| IBIS file generated by GenIBIS323.exe Version 3.23
|   TDA2x
[IBIS ver]   5.0
[File name]   TDA2x.ibs
[File Rev]   1.3.3
[Date]   Fri Sep 20, 2013, 10:27:58
[Source]   Data created at Texas Instruments
[Notes]   TDA2x 17mm IBIS Model Revision History
   TDA2x Version 1.3.3, April 21, 2016
   - Created TDA2x version from parent device
   - Does not apply to TDA2Ex device
   Version 1.3.3, September 20, 2013
   - Updated the following models to more accurately
   represent the slew and delay characteristics.
   * Models include:
   > bc1833dv40dcpbfbhhvrxp1811_sscev
   > bc1833dv40dcpbfbp1811_ssceh
   > bc1833dv40dcpbfbp1811_sscev
   > bi2c1833dvfzp18_sscev
   > iq1833dvtckpbfbp18ll_sscev
   * Peripherals that use the corresponding IO buffers
   include:
   > GPMC
   > VIN/VOUT
   > MDIO
   > RGMII
   > UART
   > McASP
   > GPIO
   > MMC
   > SPI
   > DCAN
   > I2C
   > USB (AE6)
   > Debug
   > System and Misc Signals
   Version 1.3.2, August 14, 2013
   - Updated DDR models to address the minimum supply
   voltage and the discontinuities in the vertical
   single ended models.
   Version 1.3.1, August 5, 2013
   - Updated DDR2 (1.8V) models; regenerated at 400 MHz
   Version 1.3.0, June 14, 2013
   - Added I2C models
   - Added DDR Clock pins as differential
   Version 1.2.0, May 23, 2013
   - Added DDR2 (1.8V) models
   - Added DDR DQS pins as differential
   Version 1.1.1, April 8, 2013
   - Modifications, Additions, Deletions
   * Changed name of file to be package specific
   * Updated the following source IO models:
   > DDR_SEIOPB_V
   > DDR_SEIOPB_H
   > DDR_DIFFIOPB_H
   * Replaced the following source IO models:
   > GANGARX_HMAV10GS80 with GANGARX
   > SHANTANUTX_HMAV10GS80 with
   USB3_PCIEGEN1_PCIEGEN2_TX / SATATX
   * Added the following source IO models:
   > ACSPCIE_RX
   > IHHV1833DVHYP1811_SSCEV
   > BC1833DV40DCPBFBHHVRXP1811_SSCEV
   > IQ1833DVTCKPBFBP18LL_SSCEV
   * Updated the RLC data for all pins
   * Changed the supported DDR voltage from 1.2V/1.5V
   to 1.35/1.5V for DDR3 usage
   * Updated the ball number for some signals
   Version 1.0, December 4, 2012
   - Initial Release
   Note 1) Checked by IBISCHK5.
   Note 2) Interfaces Included in this IBIS Model
   - DDR1
   - GPMC
   - VIP1
   - VIP2
   - DSS
   - HDMI1
   - RGMII
   - UART3
   - USB1
   - PCIE
   - XREFCLK
   - McASP1,2,3,4,5
   - MMC3
   - SPI1,2
   - DCAN
   - UART1,2
   - SATA1
   - I2C1
   - I2C2
[Disclaimer] Please be aware that in the absence of a written agreement,
   Texas Instruments (TI) assumes no liability for: 1) the
   accuracy of the IBIS models provided to your company, 2) the
   proper functioning of these IBIS models in your design or for
   any resulting applications, or, 3) infringement of patents,
   copyrights, or intellectual property rights resulting from
   your use of these IBIS models. TI provides IBIS models as a
   service to our customers and therefore reserves the right to
   limit distribution of the IBIS models.
[Copyright]   Property of Texas Instruments Incorporated. Unauthorised
   reproduction and/or distribution is strictly prohibited. This
   product is protected under copyright law and trade secret law
   as an unpublished work. Created 2013,(C) Copyright 2013,
   Texas Instruments Incorporated., All Rights Reserved. These
   commodities are under the U.S. Government distribution license
   control.As such,they are not to be re-exported without the
   prior approval of the U.S. Department of Commerce.
|   Component TDA2x
[Component]   TDA2x
[Manufacturer]   Texas Instruments.
| Source IO level model revisions
|Model   Revision   Date
|DDR_SEIOPB_V   2.4   14 Aug 2013
|BC1833DV40DCPBFBP1811_SSCEH   2.0   Sep 11, 2013
|DDR_SEIOPB_H   2.4   14 Aug 2013
|GANGARX   1   Sep 04, 2012
|DDR_DIFFIOPB_H   2.4   14 Aug 2013
|IQ1833DVTCKPBFBP18LL_SSCEV   2.0   Sep 11, 2013
|HDMITXPHY   0.8   Jul 12, 2011
|USB3_PCIEGEN1_PCIEGEN2_TX   1.0   Nov 07, 2012
|ACSPCIE_RX   0.5   May 16, 2012
|DDR_DIFFIOPB_V   2.4   14 Aug 2013
|BI2C1833DVFZP18_SSCEV   2.0   Sep 11, 2013
|USB2PHYCORE_HMAV10GS80   0.8   July 13, 2011
|BC1833DV40DCPBFBP1811_SSCEV   2.0   Sep 11, 2013
|BC1833DV40DCPBFBHHVRXP1811_SSCEV   2.0   Sep 11, 2013
|IHHV1833DVHYP1811_SSCEV   1.0   Dec 24, 2012
[Package]
|   typ   min   max
R_pkg   0.451804411428571   26.877E-3   1221.700E-3
L_pkg   2.34772857142857E-009 0.659E-9   5.652E-9
C_pkg   1.16282285714286E-012 0.592E-12   2.087E-12
[Pin]   signal_name   model_name   R_pin   L_pin   C_pin
Y7   ATESTV   NC
E21   DCAN1_RX   Selector_16  463.710E-3 2.345E-9   1.144E-12
E19   DCAN1_TX   Selector_16  130.950E-3 0.880E-9   0.804E-12
AC20   DDR1_A5   Selector_2   601.780E-3 2.409E-9   1.006E-12
M21   DDR1_D30   Selector_15  445.880E-3 2.447E-9   1.330E-12
P24   DDR1_DQSN3   Selector_13  461.360E-3 2.464E-9   1.164E-12
P22   DDR1_D29   Selector_15  493.080E-3 2.118E-9   1.140E-12
T24   DDR1_DQM2   Selector_17  425.130E-3 2.082E-9   1.136E-12
P21   DDR1_DQM3   Selector_17  341.520E-3 1.786E-9   1.246E-12
T25   DDR1_D23   Selector_15  416.820E-3 2.054E-9   1.079E-12
Y21   DDR1_D0   Selector_15  391.590E-3 1.635E-9   0.982E-12
U25   DDR1_DQS2   Selector_5   365.560E-3 2.080E-9   1.161E-12
R22   DDR1_D16   Selector_15  408.140E-3 2.006E-9   1.164E-12
V24   DDR1_DQSN1   Selector_13  332.830E-3 1.926E-9   1.098E-12
M25   DDR1_ECC_D0   Selector_15  615.370E-3 2.868E-9   1.361E-12
P23   DDR1_D17   Selector_15  376.150E-3 1.866E-9   1.181E-12
N24   DDR1_D26   Selector_15  465.800E-3 2.306E-9   1.305E-12
AE23   DDR1_BA2   Selector_2   668.110E-3 3.078E-9   1.348E-12
AD18   DDR1_A15   Selector_2   645.490E-3 2.726E-9   1.063E-12
AA25   DDR1_DQS0   Selector_5   355.560E-3 2.004E-9   1.041E-12
V23   DDR1_D11   Selector_15  378.670E-3 1.867E-9   1.016E-12
AD21   DDR1_WEN   Selector_2   660.220E-3 2.763E-9   1.137E-12
AC18   DDR1_CASN   Selector_2   579.300E-3 2.239E-9   1.179E-12
K23   DDR1_ECC_D4   Selector_15  623.560E-3 2.738E-9   1.233E-12
AA22   DDR1_D6   Selector_15  394.470E-3 1.827E-9   1.021E-12
AE20   DDR1_A1   Selector_2   532.570E-3 2.267E-9   1.397E-12
Y25   DDR1_D5   Selector_15  383.930E-3 2.024E-9   1.076E-12
AC21   DDR1_A4   Selector_2   645.850E-3 2.449E-9   1.255E-12
AA19   DDR1_A7   Selector_2   497.700E-3 2.270E-9   1.061E-12
R24   DDR1_D20   Selector_15  418.610E-3 2.097E-9   1.085E-12
M22   DDR1_D27   Selector_15  447.080E-3 2.390E-9   1.268E-12
K24   DDR1_DQSN_ECC   Selector_13  564.990E-3 2.914E-9   1.394E-12
AC22   DDR1_CSN0   Selector_2   637.030E-3 2.509E-9   1.304E-12
L25   DDR1_ECC_D6   Selector_15  641.400E-3 3.008E-9   1.214E-12
V22   DDR1_D12   Selector_15  385.360E-3 1.662E-9   1.016E-12
J23   DDR1_ECC_D2   Selector_15  644.370E-3 3.012E-9   1.390E-12
W22   DDR1_D9   Selector_15  388.130E-3 1.861E-9   0.929E-12
L24   DDR1_ECC_D5   Selector_15  616.230E-3 2.846E-9   1.348E-12
AA20   DDR1_DQM0   Selector_17  308.850E-3 1.445E-9   1.026E-12
AB24   DDR1_A12   Selector_2   640.730E-3 2.440E-9   1.311E-12
AB21   DDR1_VREF0   NC
AB20   DDR1_A8   Selector_2   621.390E-3 2.157E-9   1.190E-12
M24   DDR1_ECC_D1   Selector_15  635.500E-3 2.924E-9   1.360E-12
P25   DDR1_DQS3   Selector_5   465.950E-3 2.482E-9   1.310E-12
AE19   DDR1_RASN   Selector_2   604.870E-3 2.186E-9   1.440E-12
AC25   DDR1_CK   Selector_14  654.810E-3 2.979E-9   1.334E-12
U24   DDR1_DQSN2   Selector_13  347.950E-3 1.962E-9   1.148E-12
V21   DDR1_D13   Selector_15  172.230E-3 1.807E-9   1.120E-12
Y22   DDR1_D3   Selector_15  389.570E-3 1.662E-9   0.972E-12
AC23   DDR1_A6   Selector_2   646.310E-3 2.733E-9   1.343E-12
W25   DDR1_D4   Selector_15  390.500E-3 2.069E-9   1.038E-12
N22   DDR1_D31   Selector_15  439.830E-3 2.016E-9   1.110E-12
AA18   DDR1_A3   Selector_2   488.480E-3 2.281E-9   1.285E-12
N23   DDR1_D28   Selector_15  483.920E-3 2.290E-9   1.115E-12
K25   DDR1_DQS_ECC   Selector_5   573.180E-3 2.913E-9   1.379E-12
N21   DDR1_D24   Selector_15  459.010E-3 2.201E-9   1.173E-12
R25   DDR1_D19   Selector_15  417.700E-3 2.100E-9   1.051E-12
AA21   DDR1_D7   Selector_15  371.740E-3 1.559E-9   1.031E-12
AD17   DDR1_A13   Selector_2   609.270E-3 2.349E-9   1.196E-12
W21   DDR1_D8   Selector_15  394.160E-3 1.752E-9   1.125E-12
AE21   DDR1_BA1   Selector_2   642.880E-3 2.917E-9   1.281E-12
U21   DDR1_DQM1   Selector_17  274.990E-3 1.700E-9   1.008E-12
R21   DDR1_D21   Selector_15  361.860E-3 2.148E-9   1.166E-12
W24   DDR1_D2   Selector_15  385.490E-3 2.016E-9   1.030E-12
AC24   DDR1_NCK   Selector_9   652.970E-3 3.000E-9   1.347E-12
AB18   DDR1_A0   Selector_2   507.480E-3 2.394E-9   1.329E-12
AB25   DDR1_A11   Selector_2   632.080E-3 2.629E-9   1.369E-12
K22   DDR1_DQM_ECC   Selector_17  636.180E-3 2.670E-9   1.250E-12
AE17   DDR1_A14   Selector_2   619.970E-3 2.435E-9   1.045E-12
AA24   DDR1_DQSN0   Selector_13  350.870E-3 2.011E-9   0.956E-12
AD23   DDR1_ODT0   Selector_2   709.530E-3 3.055E-9   1.355E-12
N25   DDR1_D25   Selector_15  493.150E-3 2.453E-9   1.182E-12
U23   DDR1_D14   Selector_15  332.810E-3 1.858E-9   1.148E-12
AD24   DDR1_A2   Selector_2   664.380E-3 3.045E-9   1.281E-12
AB23   DDR1_A9   Selector_2   638.160E-3 2.413E-9   1.190E-12
U22   DDR1_D15   Selector_15  331.540E-3 1.705E-9   1.154E-12
T22   DDR1_D22   Selector_15  387.150E-3 1.754E-9   1.063E-12
AE18   DDR1_BA0   Selector_2   627.580E-3 2.515E-9   1.321E-12
L22   DDR1_ECC_D3   Selector_15  622.650E-3 2.631E-9   1.356E-12
T21   DDR1_D18   Selector_15  310.240E-3 1.491E-9   0.938E-12
Y24   DDR1_D1   Selector_15  379.970E-3 1.917E-9   0.986E-12
L21   DDR1_ECC_D7   Selector_15  683.310E-3 2.897E-9   1.313E-12
AB19   DDR1_CKE   Selector_2   540.190E-3 2.206E-9   0.997E-12
V25   DDR1_DQS1   Selector_5   331.770E-3 1.853E-9   1.187E-12
AB22   DDR1_A10   Selector_2   630.700E-3 2.135E-9   1.277E-12
AD20   DDR1_RST   Selector_2   668.060E-3 2.685E-9   1.312E-12
W23   DDR1_D10   Selector_15  362.420E-3 1.740E-9   0.960E-12
E20   EMU0   Selector_16  277.650E-3 1.610E-9   1.063E-12
D21   EMU1   Selector_16  479.230E-3 2.366E-9   1.180E-12
Y1   GPIO6_10   Selector_10  521.740E-3 3.084E-9   1.420E-12
W1   GPIO6_11   Selector_10  433.870E-3 2.183E-9   1.101E-12
E2   GPMC_A24   Selector_10  359.070E-3 1.975E-9   1.131E-12
D1   GPMC_A22   Selector_10  421.510E-3 2.285E-9   1.160E-12
G3   GPMC_AD9   Selector_10  421.090E-3 2.287E-9   1.339E-12
G2   GPMC_AD8   Selector_10  267.490E-3 1.834E-9   1.032E-12
N2   GPMC_A4   Selector_10  371.530E-3 2.027E-9   1.129E-12
G1   GPMC_AD2   Selector_10  320.320E-3 2.077E-9   1.172E-12
F5   GPMC_AD13   Selector_10  123.700E-3 0.854E-9   0.834E-12
K6   GPMC_A17   Selector_10  215.800E-3 1.496E-9   1.086E-12
N3   GPMC_A0   Selector_10  245.300E-3 1.481E-9   1.066E-12
L4   GPMC_A13   Selector_10  257.060E-3 1.520E-9   0.935E-12
D3   GPMC_A20   Selector_10  266.870E-3 1.817E-9   1.157E-12
M4   GPMC_A7   Selector_10  227.660E-3 1.435E-9   0.941E-12
K2   GPMC_CS3   Selector_10  402.200E-3 2.063E-9   1.291E-12
F3   GPMC_A27   Selector_10  577.110E-3 3.342E-9   1.515E-12
H4   GPMC_AD5   Selector_10  387.900E-3 2.353E-9   1.054E-12
P3   GPMC_A1   Selector_10  400.770E-3 2.018E-9   1.094E-12
L5   GPMC_A12   Selector_10  197.850E-3 1.267E-9   0.949E-12
H2   GPMC_AD3   Selector_10  184.450E-3 1.453E-9   0.953E-12
G4   GPMC_AD10   Selector_10  472.420E-3 2.631E-9   1.296E-12
H3   GPMC_AD4   Selector_10  481.420E-3 2.604E-9   1.345E-12
J3   GPMC_BEN1   Selector_10  422.980E-3 2.428E-9   1.285E-12
M5   GPMC_A6   Selector_10  230.850E-3 1.431E-9   0.974E-12
M3   GPMC_A9   Selector_10  349.820E-3 1.861E-9   0.942E-12
M6   GPMC_A10   Selector_10  290.780E-3 2.115E-9   1.176E-12
E3   GPMC_A25   Selector_10  523.900E-3 2.967E-9   1.440E-12
H6   GPMC_AD1   Selector_10  70.140E-3  0.745E-9   0.738E-12
K5   GPMC_A18   Selector_10  147.480E-3 0.958E-9   0.983E-12
M2   GPMC_BEN0   Selector_10  384.550E-3 1.923E-9   0.985E-12
J4   GPMC_AD0   Selector_10  445.610E-3 2.363E-9   1.292E-12
E5   GPMC_AD14   Selector_10  198.000E-3 1.413E-9   0.933E-12
K4   GPMC_CS0   Selector_10  246.530E-3 1.417E-9   0.920E-12
G5   GPMC_AD11   Selector_10  110.560E-3 0.844E-9   0.779E-12
G6   GPMC_AD12   Selector_10  126.070E-3 1.000E-9   0.784E-12
P1   GPMC_A2   Selector_10  533.070E-3 2.610E-9   1.250E-12
F4   GPMC_AD15   Selector_10  279.360E-3 1.630E-9   1.008E-12
L3   GPMC_A14   Selector_10  286.770E-3 1.587E-9   1.026E-12
C1   GPMC_CS1   Selector_10  425.990E-3 2.291E-9   1.117E-12
L2   GPMC_A15   Selector_10  427.460E-3 2.176E-9   1.188E-12
J5   GPMC_ADVN_ALE   Selector_10  126.710E-3 0.981E-9   0.885E-12
K1   GPMC_WAIT0   Selector_10  400.740E-3 2.102E-9   1.063E-12
D2   GPMC_A21   Selector_10  328.920E-3 1.891E-9   1.266E-12
P2   GPMC_A3   Selector_10  430.140E-3 2.168E-9   1.183E-12
E1   GPMC_A23   Selector_10  416.150E-3 2.285E-9   1.208E-12
L1   GPMC_A16   Selector_10  402.630E-3 2.104E-9   1.132E-12
M1   GPMC_A8   Selector_10  488.790E-3 2.415E-9   1.239E-12
C2   GPMC_A19   Selector_10  444.750E-3 2.652E-9   1.312E-12
F2   GPMC_WEN   Selector_10  424.150E-3 3.038E-9   1.497E-12
N6   GPMC_CLK   Selector_10  302.950E-3 1.983E-9   1.157E-12
N1   GPMC_A5   Selector_10  468.120E-3 2.440E-9   1.222E-12
E4   GPMC_A26   Selector_10  191.540E-3 1.238E-9   0.848E-12
N5   GPMC_A11   Selector_10  295.970E-3 1.733E-9   1.034E-12
H5   GPMC_AD6   Selector_10  131.890E-3 0.963E-9   0.816E-12
F1   GPMC_AD7   Selector_10  297.000E-3 1.814E-9   1.142E-12
H1   GPMC_OEN_REN   Selector_10  233.470E-3 1.955E-9   1.147E-12
K3   GPMC_CS2   Selector_10  263.620E-3 1.512E-9   0.947E-12
AE13   HDMI1_CLOCKY   Model_499   511.060E-3 3.576E-9   0.726E-12
AE14   HDMI1_DATA0Y   Model_499   449.700E-3 3.320E-9   0.646E-12
AE16   HDMI1_DATA2Y   Model_499   470.780E-3 3.387E-9   0.653E-12
AD14   HDMI1_DATA0X   Model_498   449.260E-3 3.078E-9   0.741E-12
AD16   HDMI1_DATA2X   Model_498   450.890E-3 2.959E-9   0.592E-12
AD15   HDMI1_DATA1X   Model_498   425.260E-3 2.890E-9   0.667E-12
AE15   HDMI1_DATA1Y   Model_499   463.320E-3 3.318E-9   0.738E-12
AD13   HDMI1_CLOCKX   Model_498   503.180E-3 3.217E-9   0.705E-12
G25   I2C1_SDA   Selector_7   984.150E-3 4.471E-9   1.624E-12
F23   I2C2_SCL   Selector_7   892.510E-3 3.917E-9   1.539E-12
G24   I2C1_SCL   Selector_7   1020.300E-3 4.477E-9   1.684E-12
F22   I2C2_SDA   Selector_7   802.230E-3 3.606E-9   1.632E-12
AE12   LJCB_CLKP   Model_699   427.270E-3 2.549E-9   0.759E-12
AD12   LJCB_CLKN   Model_699   399.560E-3 2.285E-9   0.821E-12
A17   MCASP1_AXR9   Selector_16  639.010E-3 3.067E-9   1.257E-12
B24   MCASP1_FSX   Selector_16  1110.900E-3 4.998E-9   1.700E-12
B15   MCASP1_AXR0   Selector_16  422.670E-3 2.198E-9   1.107E-12
C15   MCASP1_AXR14   Selector_16  253.340E-3 1.565E-9   0.933E-12
A23   MCASP1_AXR13   Selector_16  1092.300E-3 4.982E-9   1.540E-12
A15   MCASP1_AXR1   Selector_16  523.880E-3 2.560E-9   1.051E-12
A19   MCASP1_AXR10   Selector_16  779.980E-3 3.618E-9   1.389E-12
A21   MCASP1_AXR12   Selector_16  895.110E-3 4.149E-9   1.564E-12
B16   MCASP1_AXR15   Selector_16  466.140E-3 2.322E-9   1.195E-12
A16   MCASP1_AXR8   Selector_16  466.300E-3 2.392E-9   1.090E-12
A20   MCASP1_AXR11   Selector_16  890.820E-3 4.087E-9   1.607E-12
C25   MCASP1_ACLKX   Selector_16  1221.700E-3 5.206E-9   1.867E-12
B17   MCASP2_AXR3   Selector_16  518.380E-3 2.575E-9   1.145E-12
B21   MCASP2_ACLKX   Selector_16  767.630E-3 3.690E-9   1.542E-12
B20   MCASP2_FSX   Selector_16  704.240E-3 3.331E-9   1.350E-12
B23   MCASP2_AXR2   Selector_16  986.210E-3 4.307E-9   1.727E-12
C16   MCASP3_FSX   Selector_16  342.390E-3 1.864E-9   1.011E-12
C20   MCASP3_AXR1   Selector_16  742.080E-3 3.602E-9   1.505E-12
C17   MCASP3_AXR0   Selector_16  324.500E-3 1.806E-9   1.002E-12
B19   MCASP3_ACLKX   Selector_16  543.620E-3 2.687E-9   1.100E-12
D23   MCASP4_FSX   Selector_16  953.700E-3 4.218E-9   1.664E-12
E23   MCASP4_AXR1   Selector_16  1178.700E-3 5.214E-9   2.087E-12
E24   MCASP4_ACLKX   Selector_16  1218.800E-3 5.203E-9   2.019E-12
E25   MCASP4_AXR0   Selector_16  1064.300E-3 4.828E-9   1.872E-12
V2   MCASP5_AXR0   Selector_10  501.640E-3 2.583E-9   1.207E-12
W2   MCASP5_FSX   Selector_10  394.660E-3 2.073E-9   1.152E-12
V1   MCASP5_ACLKX   Selector_10  499.360E-3 2.696E-9   1.265E-12
U1   MCASP5_AXR1   Selector_10  329.480E-3 1.886E-9   1.111E-12
T1   MDIO_D   Selector_10  487.610E-3 2.629E-9   1.329E-12
R3   MDIO_MCLK   Selector_10  634.770E-3 3.175E-9   1.417E-12
W4   MMC3_CMD   Selector_10  380.060E-3 2.037E-9   1.208E-12
U5   MMC3_DAT2   Selector_10  174.080E-3 1.188E-9   1.065E-12
U6   MMC3_DAT0   Selector_10  45.368E-3  0.707E-9   0.758E-12
W3   MMC3_DAT6   Selector_10  534.640E-3 3.025E-9   1.596E-12
V3   MMC3_DAT3   Selector_10  556.770E-3 3.106E-9   1.485E-12
V4   MMC3_DAT7   Selector_10  212.570E-3 1.339E-9   0.912E-12
V6   MMC3_DAT1   Selector_10  176.740E-3 1.110E-9   1.078E-12
W5   MMC3_CLK   Selector_10  330.100E-3 2.088E-9   1.282E-12
W6   MMC3_DAT5   Selector_10  334.710E-3 2.207E-9   1.268E-12
V5   MMC3_DAT4   Selector_10  246.460E-3 1.514E-9   0.871E-12
G22   NMIN   Selector_6   798.970E-3 3.586E-9   1.571E-12
AA11   ON_OFF   Selector_18  111.570E-3 1.030E-9   0.880E-12
AE11   PCIE_TXP0   Selector_12  465.680E-3 2.523E-9   0.681E-12
AD10   PCIE_RXN0   Model_332   460.180E-3 2.608E-9   0.752E-12
AE10   PCIE_RXP0   Model_332   452.350E-3 2.692E-9   0.773E-12
AD11   PCIE_TXN0   Selector_8   456.230E-3 2.425E-9   0.719E-12
F17   PORZ   Selector_19  38.459E-3  0.727E-9   0.775E-12
H21   RESETN   Selector_6   766.440E-3 3.519E-9   1.404E-12
U3   RGMII0_RXCTL   Selector_10  399.210E-3 2.120E-9   1.010E-12
P5   RGMII0_RXD3   Selector_10  207.740E-3 1.332E-9   0.983E-12
U2   RGMII0_RXC   Selector_10  486.610E-3 2.421E-9   1.222E-12
T4   RGMII0_TXD1   Selector_10  305.720E-3 1.692E-9   1.003E-12
R6   RGMII0_TXC   Selector_10  145.130E-3 1.121E-9   0.891E-12
U4   RGMII0_RXD2   Selector_10  554.050E-3 2.804E-9   1.434E-12
T3   RGMII0_RXD1   Selector_10  465.860E-3 2.261E-9   1.169E-12
R5   RGMII0_TXD0   Selector_10  208.370E-3 1.336E-9   0.932E-12
T6   RGMII0_TXD2   Selector_10  267.640E-3 1.638E-9   1.041E-12
P6   RGMII0_TXCTL   Selector_10  33.356E-3  0.703E-9   0.782E-12
R4   RGMII0_RXD0   Selector_10  355.120E-3 1.850E-9   0.933E-12
T5   RGMII0_TXD3   Selector_10  276.180E-3 1.590E-9   1.014E-12
R2   RMII_MHZ_50_CLK   Selector_10  556.030E-3 2.883E-9   1.357E-12
G21   RSTOUTN   Selector_1   554.330E-3 2.837E-9   1.368E-12
AA13   RTC_OSC_XI_CLKIN32   NC
AA10   RTC_PORZ   Selector_19  154.820E-3 1.596E-9   1.057E-12
AA12   RTC_OSC_XO   NC
AA9   RTC_ISO   Selector_19  204.150E-3 1.944E-9   1.014E-12
D19   RTCK   Selector_1   335.270E-3 1.806E-9   1.055E-12
D22   SPI1_CS0   Selector_16  760.230E-3 3.397E-9   1.508E-12
E22   SPI1_D0   Selector_16  841.460E-3 3.816E-9   1.670E-12
C18   SPI1_SCLK   Selector_16  306.460E-3 1.707E-9   1.003E-12
C21   SPI1_D1   Selector_16  643.920E-3 2.923E-9   1.380E-12
D16   SPI1_CS1   Selector_16  220.460E-3 1.333E-9   0.935E-12
C24   SPI1_CS3   Selector_16  870.640E-3 4.054E-9   1.515E-12
C19   SPI1_CS2   Selector_16  373.120E-3 1.985E-9   1.089E-12
F25   SPI2_D1   Selector_16  1044.700E-3 4.580E-9   1.674E-12
E16   SPI2_D0   Selector_16  27.015E-3  0.667E-9   0.744E-12
D17   SPI2_CS0   Selector_16  138.970E-3 1.020E-9   0.852E-12
F24   SPI2_SCLK   Selector_16  1000.600E-3 4.289E-9   1.702E-12
E18   TCLK   Selector_3   153.370E-3 1.082E-9   0.951E-12
D20   TDI   Selector_6   384.220E-3 1.963E-9   1.093E-12
F21   TDO   Selector_1   634.310E-3 3.028E-9   1.308E-12
D18   TMS   Selector_6   152.740E-3 1.022E-9   0.961E-12
E17   TRSTN   Selector_6   26.877E-3  0.659E-9   0.750E-12
H24   UART1_RTSN   Selector_16  849.610E-3 3.946E-9   1.646E-12
H22   UART1_TXD   Selector_16  758.590E-3 3.574E-9   1.466E-12
G23   UART1_RXD   Selector_16  780.640E-3 3.621E-9   1.564E-12
H25   UART1_CTSN   Selector_16  914.490E-3 4.170E-9   1.617E-12
J24   UART2_RTSN   Selector_16  830.410E-3 3.662E-9   1.506E-12
J22   UART2_CTSN   Selector_16  648.420E-3 2.921E-9   1.361E-12
H23   UART2_RXD   Selector_16  725.070E-3 3.286E-9   1.376E-12
J25   UART2_TXD   Selector_16  858.360E-3 3.726E-9   1.657E-12
R1   UART3_RXD   Selector_10  496.020E-3 2.594E-9   1.263E-12
T2   UART3_TXD   Selector_10  526.420E-3 2.607E-9   1.235E-12
AE7   USB_TXN0   Selector_8   332.470E-3 3.109E-9   0.941E-12
AE9   USB_RXN0   Model_332   360.230E-3 2.949E-9   0.975E-12
AD9   USB_RXP0   Model_332   374.650E-3 2.983E-9   0.974E-12
AD7   USB_TXP0   Selector_12  328.260E-3 2.867E-9   1.042E-12
AE6   USB1_DRVVBUS   Selector_10  289.920E-3 1.993E-9   1.268E-12
AE8   USB1_DP   Selector_11  318.780E-3 2.432E-9   1.029E-12
AD8   USB1_DM   Selector_4   300.150E-3 2.313E-9   0.937E-12
AB1   VIN1A_D20   Selector_10  624.620E-3 3.088E-9   1.340E-12
AD6   VIN1A_FLD0   Selector_10  464.010E-3 2.293E-9   1.126E-12
AC2   VIN1A_D17   Selector_10  509.940E-3 2.553E-9   1.126E-12
Y4   VIN1A_D9   Selector_10  831.340E-3 4.527E-9   1.992E-12
Y3   VIN1A_D18   Selector_10  802.900E-3 4.088E-9   1.743E-12
AD2   VIN1A_D14   Selector_10  645.410E-3 3.060E-9   1.358E-12
AA7   VIN1A_DE0   Selector_10  151.580E-3 1.215E-9   0.961E-12
AE5   VIN1A_D1   Selector_10  512.240E-3 2.561E-9   1.241E-12
AB5   VIN1A_D6   Selector_10  393.620E-3 2.062E-9   1.098E-12
Y2   VIN1A_D23   Selector_10  476.680E-3 2.380E-9   1.137E-12
AE3   VIN1A_D10   Selector_10  664.240E-3 3.141E-9   1.411E-12
AA6   VIN1B_CLK1   Selector_10  146.440E-3 1.089E-9   0.829E-12
AB3   VIN1A_D15   Selector_10  391.110E-3 2.132E-9   1.071E-12
AB7   VIN1A_D4   Selector_10  615.840E-3 3.507E-9   1.543E-12
AA2   VIN1A_D16   Selector_10  370.670E-3 2.037E-9   1.060E-12
AD3   VIN1A_D12   Selector_10  542.380E-3 2.707E-9   1.175E-12
AC5   VIN1A_VSYNC0   Selector_10  362.920E-3 1.987E-9   1.115E-12
AB6   VIN1A_CLK0   Selector_10  272.590E-3 1.562E-9   0.914E-12
AA4   VIN1A_D11   Selector_10  348.230E-3 1.856E-9   1.112E-12
Y5   VIN1A_D3   Selector_10  164.710E-3 1.061E-9   0.819E-12
AA1   VIN1A_D22   Selector_10  494.950E-3 2.385E-9   1.290E-12
AA5   VIN1A_D2   Selector_10  203.590E-3 1.333E-9   0.897E-12
AC1   VIN1A_D21   Selector_10  529.070E-3 2.930E-9   1.371E-12
AD4   VIN1A_D7   Selector_10  643.120E-3 2.989E-9   1.439E-12
AC3   VIN1A_D13   Selector_10  528.880E-3 2.760E-9   1.179E-12
AC6   VIN1A_HSYNC0   Selector_10  334.690E-3 1.796E-9   1.054E-12
AB2   VIN1A_D19   Selector_10  683.400E-3 3.260E-9   1.503E-12
AD5   VIN1A_D0   Selector_10  492.990E-3 2.517E-9   1.248E-12
AA3   VIN1A_D8   Selector_10  242.030E-3 1.438E-9   0.961E-12
AE4   VIN1A_D5   Selector_10  583.240E-3 2.760E-9   1.314E-12
B4   VIN2A_DE0   Selector_16  497.810E-3 2.562E-9   1.390E-12
D5   VIN2A_HSYNC0   Selector_16  138.660E-3 0.948E-9   0.779E-12
B6   VIN2A_D11   Selector_16  340.620E-3 1.891E-9   0.949E-12
B3   VIN2A_D3   Selector_16  373.680E-3 2.049E-9   1.130E-12
B8   VIN2A_D17   Selector_16  308.300E-3 1.836E-9   1.031E-12
D8   VIN2A_D21   Selector_16  172.190E-3 1.187E-9   0.815E-12
A8   VIN2A_D18   Selector_16  349.990E-3 2.016E-9   1.092E-12
B5   VIN2A_D7   Selector_16  113.830E-3 1.275E-9   0.955E-12
C4   VIN2A_VSYNC0   Selector_16  442.750E-3 2.475E-9   1.196E-12
F8   VIN2A_D22   Selector_16  34.135E-3  0.753E-9   0.793E-12
D6   VIN2A_D15   Selector_16  177.900E-3 1.312E-9   0.954E-12
E8   VIN2A_D12   Selector_16  35.490E-3  0.788E-9   0.852E-12
A3   VIN2A_D4   Selector_16  322.430E-3 1.992E-9   1.253E-12
D7   VIN2A_D19   Selector_16  216.070E-3 1.428E-9   0.983E-12
A6   VIN2A_D13   Selector_16  342.780E-3 1.964E-9   1.151E-12
A4   VIN2A_D6   Selector_16  398.920E-3 2.267E-9   1.141E-12
D4   VIN2A_CLK0   Selector_16  334.400E-3 1.910E-9   1.068E-12
C8   VIN2A_D20   Selector_16  305.840E-3 1.772E-9   1.053E-12
C6   VIN2A_D5   Selector_16  492.200E-3 2.818E-9   1.363E-12
E9   VIN2A_D23   Selector_16  89.939E-3  0.866E-9   0.806E-12
B2   VIN2A_D1   Selector_16  381.890E-3 2.351E-9   1.097E-12
C5   VIN2A_D8   Selector_16  404.700E-3 2.266E-9   1.350E-12
E7   VIN2A_D2   Selector_16  50.536E-3  0.781E-9   0.799E-12
A5   VIN2A_D10   Selector_16  242.060E-3 1.967E-9   1.141E-12
E6   VIN2A_FLD0   Selector_16  274.220E-3 1.791E-9   1.304E-12
B7   VIN2A_D16   Selector_16  338.760E-3 1.841E-9   0.930E-12
A7   VIN2A_D9   Selector_16  266.920E-3 1.701E-9   1.069E-12
C3   VIN2A_D0   Selector_16  353.730E-3 2.020E-9   1.142E-12
C7   VIN2A_D14   Selector_16  205.720E-3 1.340E-9   0.945E-12
A11   VOUT1_D2   Selector_16  414.210E-3 2.319E-9   1.034E-12
E13   VOUT1_VSYNC   Selector_16  252.020E-3 1.772E-9   1.046E-12
D14   VOUT1_D22   Selector_16  425.030E-3 2.364E-9   1.243E-12
C13   VOUT1_D15   Selector_16  543.860E-3 2.696E-9   1.359E-12
B14   VOUT1_D6   Selector_16  713.520E-3 3.538E-9   1.520E-12
E15   VOUT1_D19   Selector_16  442.740E-3 2.979E-9   1.379E-12
D11   VOUT1_D23   Selector_16  151.680E-3 1.114E-9   0.941E-12
E12   VOUT1_HSYNC   Selector_16  179.020E-3 1.228E-9   0.898E-12
A10   VOUT1_D14   Selector_16  506.430E-3 2.691E-9   1.293E-12
B9   VOUT1_D0   Selector_16  268.920E-3 1.610E-9   1.022E-12
E14   VOUT1_D21   Selector_16  358.380E-3 2.313E-9   1.156E-12
C14   VOUT1_D12   Selector_16  488.910E-3 2.694E-9   1.318E-12
B11   VOUT1_D9   Selector_16  409.280E-3 2.026E-9   1.193E-12
D9   VOUT1_D20   Selector_16  185.090E-3 1.275E-9   0.804E-12
A12   VOUT1_D5   Selector_16  533.490E-3 2.658E-9   1.286E-12
C10   VOUT1_D13   Selector_16  270.190E-3 1.514E-9   0.854E-12
A9   VOUT1_D1   Selector_16  384.810E-3 2.063E-9   0.966E-12
D15   VOUT1_D18   Selector_16  515.610E-3 2.997E-9   1.399E-12
D10   VOUT1_CLK   Selector_16  108.040E-3 0.846E-9   0.755E-12
A14   VOUT1_D8   Selector_16  717.820E-3 3.276E-9   1.246E-12
A13   VOUT1_D4   Selector_16  574.670E-3 2.900E-9   1.311E-12
C9   VOUT1_D3   Selector_16  259.750E-3 1.574E-9   0.931E-12
E10   VOUT1_D17   Selector_16  27.061E-3  0.667E-9   0.678E-12
C11   VOUT1_D16   Selector_16  352.470E-3 1.812E-9   1.038E-12
E11   VOUT1_FLD   Selector_16  98.068E-3  0.849E-9   0.810E-12
D13   VOUT1_DE   Selector_16  332.020E-3 1.846E-9   1.152E-12
B12   VOUT1_D10   Selector_16  536.060E-3 2.568E-9   1.259E-12
B10   VOUT1_D11   Selector_16  354.910E-3 1.895E-9   1.036E-12
B13   VOUT1_D7   Selector_16  637.340E-3 2.955E-9   1.264E-12
AA16   WAKEUP0   Selector_19  915.000E-3 5.652E-9   1.490E-12
AA17   WAKEUP1   Selector_19  926.080E-3 4.252E-9   1.553E-12
AB17   WAKEUP2   Selector_19  883.760E-3 4.103E-9   1.486E-12
AC17   WAKEUP3   Selector_19  908.090E-3 4.114E-9   1.552E-12
AC13   XI_OSC1   NC
AC14   XI_OSC0   NC
AB14   XO_OSC0   NC
AB13   XO_OSC1   NC
C23   XREF_CLK0   Selector_16  892.740E-3 4.011E-9   1.463E-12
C22   XREF_CLK1   Selector_16  804.240E-3 3.591E-9   1.533E-12
[Diff Pin] inv_pin vdiff tdelay_typ tdelay_min tdelay_max
|Differential signal data for cell USB3_PCIEGEN1_PCIEGEN2_TX
|PCIE_TXP0   PCIE_TXN0
AE11   AD11   200m   0
|USB_TXP0   USB_TXN0
AD7   AE7   200m   0
|Differential signal data for cell HDMITXPHY
|HDMI1_DATA0X   HDMI1_DATA0Y
AD14   AE14   0.0V   0.0s
|HDMI1_DATA2X   HDMI1_DATA2Y
AD16   AE16   0.0V   0.0s
|HDMI1_CLOCKX   HDMI1_CLOCKY
AD13   AE13   0.0V   0.0s
|HDMI1_DATA1X   HDMI1_DATA1Y
AD15   AE15   0.0V   0.0s
|Differential signal data for cell ACSPCIE_RX
|LJCB_CLKP   LJCB_CLKN
AE12   AD12   150m   NA   NA   NA
|Differential signal data for cell DDR_DIFFIOPB_V
|DDR1_CK   DDR1_NCK
AC25   AC24   200m   0
|Differential signal data for cell USB2PHYCORE_HMAV10GS80
|USB1_DP   USB1_DM
AE8   AD8   200mV 0ns 0ns 0ns
|Differential signal data for cell GANGARX
|PCIE_RXP0   PCIE_RXN0
AE10   AD10   100mV  NA
|USB_RXP0   USB_RXN0
AD9   AE9   100mV  NA
|Differential signal data for cell DDR_DIFFIOPB_H
|DDR1_DQS0   DDR1_DQSN0
AA25   AA24   200m   0
|DDR1_DQS3   DDR1_DQSN3
P25   P24   200m   0
|DDR1_DQS_ECC   DDR1_DQSN_ECC
K25   K24   200m   0
|DDR1_DQS1   DDR1_DQSN1
V25   V24   200m   0
|DDR1_DQS2   DDR1_DQSN2
U25   U24   200m   0
|   Usage OUTPUT#1.8/3.3###BC1833DV40DCPBFBP1811_SSCEV.PAD
|   Base model BC1833DV40DCPBFBP1811_SSCEV
[Model Selector] Selector_1
Model_704 I/O,1.8V,40D CLASS MODE FAST MODE,IND,10 PERCENT%,BC40D_V_10P_!SC1_1P8
Model_705 I/O,1.8V,40C CLASS MODE SLOW MODE,IND,10 PERCENT%,BC40D_V_10P_SC1_1P8
Model_706 I/O,1.8V,40D CLASS MODE FAST MODE,IND,5 PERCENT%,BC40D_V_5P_!SC1_1P8
Model_707 I/O,1.8V,40C CLASS MODE SLOW MODE,IND,5 PERCENT%,BC40D_V_5P_SC1_1P8
Model_708 I/O,3.3V,40D CLASS MODE FAST MODE,IND,10 PERCENT%,BC40D_V_10P_!SC1_3P3
Model_709 I/O,3.3V,40C CLASS MODE SLOW MODE,IND,10 PERCENT%,BC40D_V_10P_SC1_3P3
Model_710 I/O,3.3V,40D CLASS MODE FAST MODE,IND,5 PERCENT%,BC40D_V_5P_!SC1_3P3
Model_711 I/O,3.3V,40C CLASS MODE SLOW MODE,IND,5 PERCENT%,BC40D_V_5P_SC1_3P3
|   Usage OUTPUT#1.35/1.5/1.8###DDR_SEIOPB_V.PAD
|   Base model DDR_SEIOPB_V
[Model Selector] Selector_2
Model_100 I/O,1.8V,SR100_DRV34_1P8
Model_101 I/O,1.8V,SR110_DRV34_1P8
Model_102 I/O,1.8V,SR111_DRV34_1P8
Model_103 I/O,1.8V,SR001_DRV34_1P8
Model_104 I/O,1.8V,SR000_DRV34_1P8
Model_114 I/O,1.5V,SR011_DRV40_1P5
Model_115 I/O,1.5V,SR010_DRV40_1P5
Model_116 I/O,1.5V,SR101_DRV40_1P5
Model_117 I/O,1.5V,SR100_DRV40_1P5
Model_118 I/O,1.5V,SR110_DRV40_1P5
Model_119 I/O,1.5V,SR111_DRV40_1P5
Model_120 I/O,1.5V,SR001_DRV40_1P5
Model_121 I/O,1.5V,SR000_DRV40_1P5
Model_122 I/O,1.5V,SR011_DRV34_1P5
Model_123 I/O,1.5V,SR010_DRV34_1P5
Model_124 I/O,1.5V,SR101_DRV34_1P5
Model_125 I/O,1.5V,SR100_DRV34_1P5
Model_126 I/O,1.5V,SR110_DRV34_1P5
Model_127 I/O,1.5V,SR111_DRV34_1P5
Model_128 I/O,1.5V,SR001_DRV34_1P5
Model_129 I/O,1.5V,SR000_DRV34_1P5
Model_130 I/O,1.5V,SR011_DRV48_1P5
Model_131 I/O,1.5V,SR010_DRV48_1P5
Model_132 I/O,1.5V,SR101_DRV48_1P5
Model_133 I/O,1.5V,SR100_DRV48_1P5
Model_134 I/O,1.5V,SR110_DRV48_1P5
Model_135 I/O,1.5V,SR111_DRV48_1P5
Model_136 I/O,1.5V,SR001_DRV48_1P5
Model_137 I/O,1.5V,SR000_DRV48_1P5
Model_138 I/O,1.35V,SR011_DRV40_1P35
Model_139 I/O,1.35V,SR010_DRV40_1P35
Model_140 I/O,1.35V,SR101_DRV40_1P35
Model_141 I/O,1.35V,SR100_DRV40_1P35
Model_142 I/O,1.35V,SR110_DRV40_1P35
Model_143 I/O,1.35V,SR111_DRV40_1P35
Model_144 I/O,1.35V,SR001_DRV40_1P35
Model_145 I/O,1.35V,SR000_DRV40_1P35
Model_146 I/O,1.35V,SR011_DRV34_1P35
Model_147 I/O,1.35V,SR010_DRV34_1P35
Model_148 I/O,1.35V,SR101_DRV34_1P35
Model_149 I/O,1.35V,SR100_DRV34_1P35
Model_150 I/O,1.35V,SR110_DRV34_1P35
Model_151 I/O,1.35V,SR111_DRV34_1P35
Model_152 I/O,1.35V,SR001_DRV34_1P35
Model_153 I/O,1.35V,SR000_DRV34_1P35
Model_154 I/O,1.35V,SR011_DRV48_1P35
Model_155 I/O,1.35V,SR010_DRV48_1P35
Model_156 I/O,1.35V,SR101_DRV48_1P35
Model_157 I/O,1.35V,SR100_DRV48_1P35
Model_158 I/O,1.35V,SR110_DRV48_1P35
Model_159 I/O,1.35V,SR111_DRV48_1P35
Model_160 I/O,1.35V,SR001_DRV48_1P35
Model_161 I/O,1.35V,SR000_DRV48_1P35
Model_81 I/O,1.8V,SR011_DRV48_1P8
Model_82 I/O,1.8V,SR010_DRV48_1P8
Model_83 I/O,1.8V,SR101_DRV48_1P8
Model_84 I/O,1.8V,SR100_DRV48_1P8
Model_85 I/O,1.8V,SR110_DRV48_1P8
Model_86 I/O,1.8V,SR111_DRV48_1P8
Model_87 I/O,1.8V,SR001_DRV48_1P8
Model_88 I/O,1.8V,SR000_DRV48_1P8
Model_89 I/O,1.8V,SR011_DRV40_1P8
Model_90 I/O,1.8V,SR010_DRV40_1P8
Model_91 I/O,1.8V,SR101_DRV40_1P8
Model_92 I/O,1.8V,SR100_DRV40_1P8
Model_93 I/O,1.8V,SR110_DRV40_1P8
Model_94 I/O,1.8V,SR111_DRV40_1P8
Model_95 I/O,1.8V,SR001_DRV40_1P8
Model_96 I/O,1.8V,SR000_DRV40_1P8
Model_97 I/O,1.8V,SR011_DRV34_1P8
Model_98 I/O,1.8V,SR010_DRV34_1P8
Model_99 I/O,1.8V,SR101_DRV34_1P8
|   Usage INPUT#1.8/3.3###IQ1833DVTCKPBFBP18LL_SSCEV.PAD
|   Base model IQ1833DVTCKPBFBP18LL_SSCEV
[Model Selector] Selector_3
Model_494 INPUT,1.8V,1.8V MODE,IND,10 PERCENT%,IQ1833_V_10P_1P8
Model_495 INPUT,1.8V,1.8V MODE,IND,5 PERCENT%,IQ1833_V_5P_1P8
Model_496 INPUT,3.3V,3.3V MODE,IND,10 PERCENT%,IQ1833_V_10P_3P3
Model_497 INPUT,3.3V,3.3V MODE,IND,5 PERCENT%,IQ1833_V_5P_3P3
|   Usage I/O#X###USB2PHYCORE_HMAV10GS80.DM
|   Base model USB2PHYCORE_HMAV10GS80
[Model Selector] Selector_4
Model_713 3-STATE,3.3000V,fsdm_tx
Model_715 3-STATE,3.3000V,lsdm_50pf_tx
Model_717 3-STATE,3.3000V,lsdm_200pf_tx
Model_719 3-STATE,3.3000V,lsdm_400pf_tx
Model_721 3-STATE,3.3000V,lsdm_600pf_tx
Model_722 INPUT,3.3V,fsrx
Model_724 3-STATE,0.8000V,hsdm_tx
Model_725 INPUT,3.3V,hsrx
|   Usage I/O#1.35/1.5/1.8###DDR_DIFFIOPB_H.PADP
|   Base model DDR_DIFFIOPB_H
[Model Selector] Selector_5
Model_413 I/O,1.8V,SR011_DRV48_1P8
Model_414 I/O,1.8V,SR010_DRV48_1P8
Model_415 I/O,1.8V,SR101_DRV48_1P8
Model_416 I/O,1.8V,SR100_DRV48_1P8
Model_417 I/O,1.8V,SR110_DRV48_1P8
Model_418 I/O,1.8V,SR111_DRV48_1P8
Model_419 I/O,1.8V,SR001_DRV48_1P8
Model_420 I/O,1.8V,SR000_DRV48_1P8
Model_421 I/O,1.8V,SR011_DRV40_1P8
Model_422 I/O,1.8V,SR010_DRV40_1P8
Model_423 I/O,1.8V,SR101_DRV40_1P8
Model_424 I/O,1.8V,SR100_DRV40_1P8
Model_425 I/O,1.8V,SR110_DRV40_1P8
Model_426 I/O,1.8V,SR111_DRV40_1P8
Model_427 I/O,1.8V,SR001_DRV40_1P8
Model_428 I/O,1.8V,SR000_DRV40_1P8
Model_429 I/O,1.8V,SR011_DRV34_1P8
Model_430 I/O,1.8V,SR010_DRV34_1P8
Model_431 I/O,1.8V,SR101_DRV34_1P8
Model_432 I/O,1.8V,SR100_DRV34_1P8
Model_433 I/O,1.8V,SR110_DRV34_1P8
Model_434 I/O,1.8V,SR111_DRV34_1P8
Model_435 I/O,1.8V,SR001_DRV34_1P8
Model_436 I/O,1.8V,SR000_DRV34_1P8
Model_437 INPUT,1.5V,DDR3_ODT_80_1P5
Model_438 INPUT,1.5V,DDR3_ODT_60_1P5
Model_439 INPUT,1.5V,DDR3_ODT_120_1P5
Model_440 INPUT,1.35V,DDR3L_ODT_80_1P35
Model_441 INPUT,1.35V,DDR3L_ODT_60_1P35
Model_442 INPUT,1.35V,DDR3L_ODT_120_1P35
Model_443 INPUT,1.8V,DDR2_ODT_120_1P8
Model_444 INPUT,1.8V,DDR2_ODT_80_1P8
Model_445 INPUT,1.8V,DDR2_ODT_60_1P8
Model_446 I/O,1.5V,SR011_DRV40_1P5
Model_447 I/O,1.5V,SR010_DRV40_1P5
Model_448 I/O,1.5V,SR101_DRV40_1P5
Model_449 I/O,1.5V,SR100_DRV40_1P5
Model_450 I/O,1.5V,SR110_DRV40_1P5
Model_451 I/O,1.5V,SR111_DRV40_1P5
Model_452 I/O,1.5V,SR001_DRV40_1P5
Model_453 I/O,1.5V,SR000_DRV40_1P5
Model_454 I/O,1.5V,SR011_DRV34_1P5
Model_455 I/O,1.5V,SR010_DRV34_1P5
Model_456 I/O,1.5V,SR101_DRV34_1P5
Model_457 I/O,1.5V,SR100_DRV34_1P5
Model_458 I/O,1.5V,SR110_DRV34_1P5
Model_459 I/O,1.5V,SR111_DRV34_1P5
Model_460 I/O,1.5V,SR001_DRV34_1P5
Model_461 I/O,1.5V,SR000_DRV34_1P5
Model_462 I/O,1.5V,SR011_DRV48_1P5
Model_463 I/O,1.5V,SR010_DRV48_1P5
Model_464 I/O,1.5V,SR101_DRV48_1P5
Model_465 I/O,1.5V,SR100_DRV48_1P5
Model_466 I/O,1.5V,SR110_DRV48_1P5
Model_467 I/O,1.5V,SR111_DRV48_1P5
Model_468 I/O,1.5V,SR001_DRV48_1P5
Model_469 I/O,1.5V,SR000_DRV48_1P5
Model_470 I/O,1.35V,SR011_DRV40_1P35
Model_471 I/O,1.35V,SR010_DRV40_1P35
Model_472 I/O,1.35V,SR101_DRV40_1P35
Model_473 I/O,1.35V,SR100_DRV40_1P35
Model_474 I/O,1.35V,SR110_DRV40_1P35
Model_475 I/O,1.35V,SR111_DRV40_1P35
Model_476 I/O,1.35V,SR001_DRV40_1P35
Model_477 I/O,1.35V,SR000_DRV40_1P35
Model_478 I/O,1.35V,SR011_DRV34_1P35
Model_479 I/O,1.35V,SR010_DRV34_1P35
Model_480 I/O,1.35V,SR101_DRV34_1P35
Model_481 I/O,1.35V,SR100_DRV34_1P35
Model_482 I/O,1.35V,SR110_DRV34_1P35
Model_483 I/O,1.35V,SR111_DRV34_1P35
Model_484 I/O,1.35V,SR001_DRV34_1P35
Model_485 I/O,1.35V,SR000_DRV34_1P35
Model_486 I/O,1.35V,SR011_DRV48_1P35
Model_487 I/O,1.35V,SR010_DRV48_1P35
Model_488 I/O,1.35V,SR101_DRV48_1P35
Model_489 I/O,1.35V,SR100_DRV48_1P35
Model_490 I/O,1.35V,SR110_DRV48_1P35
Model_491 I/O,1.35V,SR111_DRV48_1P35
Model_492 I/O,1.35V,SR001_DRV48_1P35
Model_493 I/O,1.35V,SR000_DRV48_1P35
|   Usage INPUT#1.8/3.3###BC1833DV40DCPBFBP1811_SSCEV.PAD
|   Base model BC1833DV40DCPBFBP1811_SSCEV
[Model Selector] Selector_6
Model_704 I/O,1.8V,40D CLASS MODE FAST MODE,IND,10 PERCENT%,BC40D_V_10P_!SC1_1P8
Model_705 I/O,1.8V,40C CLASS MODE SLOW MODE,IND,10 PERCENT%,BC40D_V_10P_SC1_1P8
Model_706 I/O,1.8V,40D CLASS MODE FAST MODE,IND,5 PERCENT%,BC40D_V_5P_!SC1_1P8
Model_707 I/O,1.8V,40C CLASS MODE SLOW MODE,IND,5 PERCENT%,BC40D_V_5P_SC1_1P8
Model_708 I/O,3.3V,40D CLASS MODE FAST MODE,IND,10 PERCENT%,BC40D_V_10P_!SC1_3P3
Model_709 I/O,3.3V,40C CLASS MODE SLOW MODE,IND,10 PERCENT%,BC40D_V_10P_SC1_3P3
Model_710 I/O,3.3V,40D CLASS MODE FAST MODE,IND,5 PERCENT%,BC40D_V_5P_!SC1_3P3
Model_711 I/O,3.3V,40C CLASS MODE SLOW MODE,IND,5 PERCENT%,BC40D_V_5P_SC1_3P3
|   Usage I/O#1.8/3.3###BI2C1833DVFZP18_SSCEV.PAD
|   Base model BI2C1833DVFZP18_SSCEV
[Model Selector] Selector_7
Model_700 I/O_OPEN_DRAIN,1.8V,FAST MODE AND STD MODE,IND,10 PERCENT%,FAST_STD_MODE_1.8V_10P_1P8
Model_701 I/O_OPEN_DRAIN,3.3V,FAST MODE AND STD MODE,IND,10 PERCENT%,FAST_STD_MODE_3.3V_10P_3P3
Model_702 I/O_OPEN_DRAIN,1.8V,FAST MODE AND STD MODE,IND,5 PERCENT%,FAST_STD_MODE_1.8V_5P_1P8
Model_703 I/O_OPEN_DRAIN,3.3V,FAST MODE AND STD MODE,IND,5 PERCENT%,FAST_STD_MODE_3.3V_5P_3P3
|   Usage OUTPUT#X###USB3_PCIEGEN1_PCIEGEN2_TX.TXN
|   Base model USB3_PCIEGEN1_PCIEGEN2_TX
[Model Selector] Selector_8
Model_500 3-STATE,1.1V,USB3_TX_FS_NO_DEEMPHASIS
Model_501 3-STATE,1.1V,USB3_TX_FS_3p5_DEEMPHASIS
Model_502 3-STATE,1.1V,USB3_TX_HS_NO_DEEMPHASIS
Model_503 3-STATE,1.1V,PCIEGEN1_TX_FS_NO_DEEMPHASIS_1p2v
Model_504 3-STATE,1.1V,PCIEGEN1_TX_FS_NO_DEEMPHASIS_0p8v
Model_505 3-STATE,1.1V,PCIEGEN1_TX_FS_NO_DEEMPHASIS_0p6v
Model_506 3-STATE,1.1V,PCIEGEN1_TX_FS_NO_DEEMPHASIS_0p4v
Model_507 3-STATE,1.1V,PCIEGEN1_TX_FS_3p5_DEEMPHASIS_1p2v
Model_508 3-STATE,1.1V,PCIEGEN1_TX_FS_3p5_DEEMPHASIS_0p8v
Model_509 3-STATE,1.1V,PCIEGEN1_TX_FS_3p5_DEEMPHASIS_0p6v
Model_510 3-STATE,1.1V,PCIEGEN1_TX_FS_3p5_DEEMPHASIS_0p4v
Model_511 3-STATE,1.1V,PCIEGEN1_TX_HS_NO_DEEMPHASIS_0p6v
Model_512 3-STATE,1.1V,PCIEGEN1_TX_HS_NO_DEEMPHASIS_0p4v
Model_513 3-STATE,1.1V,PCIEGEN1_TX_HS_NO_DEEMPHASIS_0p3v
Model_514 3-STATE,1.1V,PCIEGEN1_TX_HS_NO_DEEMPHASIS_0p2v
Model_515 3-STATE,1.1V,PCIEGEN2_TX_FS_NO_DEEMPHASIS_1p2v
Model_516 3-STATE,1.1V,PCIEGEN2_TX_FS_NO_DEEMPHASIS_0p8v
Model_517 3-STATE,1.1V,PCIEGEN2_TX_FS_NO_DEEMPHASIS_0p6v
Model_518 3-STATE,1.1V,PCIEGEN2_TX_FS_NO_DEEMPHASIS_0p4v
Model_519 3-STATE,1.1V,PCIEGEN2_TX_FS_3p5_DEEMPHASIS_1p2v
Model_520 3-STATE,1.1V,PCIEGEN2_TX_FS_3p5_DEEMPHASIS_0p8v
Model_521 3-STATE,1.1V,PCIEGEN2_TX_FS_3p5_DEEMPHASIS_0p6v
Model_522 3-STATE,1.1V,PCIEGEN2_TX_FS_3p5_DEEMPHASIS_0p4v
Model_523 3-STATE,1.1V,PCIEGEN2_TX_FS_6p0_DEEMPHASIS_1p2v
Model_524 3-STATE,1.1V,PCIEGEN2_TX_FS_6p0_DEEMPHASIS_0p8v
Model_525 3-STATE,1.1V,PCIEGEN2_TX_FS_6p0_DEEMPHASIS_0p6v
Model_526 3-STATE,1.1V,PCIEGEN2_TX_FS_6p0_DEEMPHASIS_0p4v
Model_527 3-STATE,1.1V,PCIEGEN2_TX_HS_NO_DEEMPHASIS_0p6v
Model_528 3-STATE,1.1V,PCIEGEN2_TX_HS_NO_DEEMPHASIS_0p4v
Model_529 3-STATE,1.1V,PCIEGEN2_TX_HS_NO_DEEMPHASIS_0p3v
Model_530 3-STATE,1.1V,PCIEGEN2_TX_HS_NO_DEEMPHASIS_0p2v
|   Usage OUTPUT#1.35/1.5/1.8###DDR_DIFFIOPB_V.PADN
|   Base model DDR_DIFFIOPB_V
[Model Selector] Selector_9
Model_618 I/O,1.8V,SR011_DRV48_1P8
Model_619 I/O,1.8V,SR010_DRV48_1P8
Model_620 I/O,1.8V,SR101_DRV48_1P8
Model_621 I/O,1.8V,SR100_DRV48_1P8
Model_622 I/O,1.8V,SR110_DRV48_1P8
Model_623 I/O,1.8V,SR111_DRV48_1P8
Model_624 I/O,1.8V,SR001_DRV48_1P8
Model_625 I/O,1.8V,SR000_DRV48_1P8
Model_626 I/O,1.8V,SR011_DRV40_1P8
Model_627 I/O,1.8V,SR010_DRV40_1P8
Model_628 I/O,1.8V,SR101_DRV40_1P8
Model_629 I/O,1.8V,SR100_DRV40_1P8
Model_630 I/O,1.8V,SR110_DRV40_1P8
Model_631 I/O,1.8V,SR111_DRV40_1P8
Model_632 I/O,1.8V,SR001_DRV40_1P8
Model_633 I/O,1.8V,SR000_DRV40_1P8
Model_634 I/O,1.8V,SR011_DRV34_1P8
Model_635 I/O,1.8V,SR010_DRV34_1P8
Model_636 I/O,1.8V,SR101_DRV34_1P8
Model_637 I/O,1.8V,SR100_DRV34_1P8
Model_638 I/O,1.8V,SR110_DRV34_1P8
Model_639 I/O,1.8V,SR111_DRV34_1P8
Model_640 I/O,1.8V,SR001_DRV34_1P8
Model_641 I/O,1.8V,SR000_DRV34_1P8
Model_651 I/O,1.5V,SR011_DRV40_1P5
Model_652 I/O,1.5V,SR010_DRV40_1P5
Model_653 I/O,1.5V,SR101_DRV40_1P5
Model_654 I/O,1.5V,SR100_DRV40_1P5
Model_655 I/O,1.5V,SR110_DRV40_1P5
Model_656 I/O,1.5V,SR111_DRV40_1P5
Model_657 I/O,1.5V,SR001_DRV40_1P5
Model_658 I/O,1.5V,SR000_DRV40_1P5
Model_659 I/O,1.5V,SR011_DRV34_1P5
Model_660 I/O,1.5V,SR010_DRV34_1P5
Model_661 I/O,1.5V,SR101_DRV34_1P5
Model_662 I/O,1.5V,SR100_DRV34_1P5
Model_663 I/O,1.5V,SR110_DRV34_1P5
Model_664 I/O,1.5V,SR111_DRV34_1P5
Model_665 I/O,1.5V,SR001_DRV34_1P5
Model_666 I/O,1.5V,SR000_DRV34_1P5
Model_667 I/O,1.5V,SR011_DRV48_1P5
Model_668 I/O,1.5V,SR010_DRV48_1P5
Model_669 I/O,1.5V,SR101_DRV48_1P5
Model_670 I/O,1.5V,SR100_DRV48_1P5
Model_671 I/O,1.5V,SR110_DRV48_1P5
Model_672 I/O,1.5V,SR111_DRV48_1P5
Model_673 I/O,1.5V,SR001_DRV48_1P5
Model_674 I/O,1.5V,SR000_DRV48_1P5
Model_675 I/O,1.35V,SR011_DRV40_1P35
Model_676 I/O,1.35V,SR010_DRV40_1P35
Model_677 I/O,1.35V,SR101_DRV40_1P35
Model_678 I/O,1.35V,SR100_DRV40_1P35
Model_679 I/O,1.35V,SR110_DRV40_1P35
Model_680 I/O,1.35V,SR111_DRV40_1P35
Model_681 I/O,1.35V,SR001_DRV40_1P35
Model_682 I/O,1.35V,SR000_DRV40_1P35
Model_683 I/O,1.35V,SR011_DRV34_1P35
Model_684 I/O,1.35V,SR010_DRV34_1P35
Model_685 I/O,1.35V,SR101_DRV34_1P35
Model_686 I/O,1.35V,SR100_DRV34_1P35
Model_687 I/O,1.35V,SR110_DRV34_1P35
Model_688 I/O,1.35V,SR111_DRV34_1P35
Model_689 I/O,1.35V,SR001_DRV34_1P35
Model_690 I/O,1.35V,SR000_DRV34_1P35
Model_691 I/O,1.35V,SR011_DRV48_1P35
Model_692 I/O,1.35V,SR010_DRV48_1P35
Model_693 I/O,1.35V,SR101_DRV48_1P35
Model_694 I/O,1.35V,SR100_DRV48_1P35
Model_695 I/O,1.35V,SR110_DRV48_1P35
Model_696 I/O,1.35V,SR111_DRV48_1P35
Model_697 I/O,1.35V,SR001_DRV48_1P35
Model_698 I/O,1.35V,SR000_DRV48_1P35
|   Usage I/O#1.8/3.3###BC1833DV40DCPBFBP1811_SSCEH.PAD
|   Base model BC1833DV40DCPBFBP1811_SSCEH
[Model Selector] Selector_10
Model_323 I/O,1.8V,40D CLASS MODE FAST MODE,IND,10 PERCENT%,BC40D_H_10P_!SC1_1P8
Model_324 I/O,1.8V,40C CLASS MODE SLOW MODE,IND,10 PERCENT%,BC40D_H_10P_SC1_1P8
Model_325 I/O,1.8V,40D CLASS MODE FAST MODE,IND,5 PERCENT%,BC40D_H_5P_!SC1_1P8
Model_326 I/O,1.8V,40C CLASS MODE SLOW MODE,IND,5 PERCENT%,BC40D_H_5P_SC1_1P8
Model_327 I/O,3.3V,40D CLASS MODE FAST MODE,IND,10 PERCENT%,BC40D_H_10P_!SC1_3P3
Model_328 I/O,3.3V,40C CLASS MODE SLOW MODE,IND,10 PERCENT%,BC40D_H_10P_SC1_3P3
Model_329 I/O,3.3V,40D CLASS MODE FAST MODE,IND,5 PERCENT%,BC40D_H_5P_!SC1_3P3
Model_330 I/O,3.3V,40C CLASS MODE SLOW MODE,IND,5 PERCENT%,BC40D_H_5P_SC1_3P3
|   Usage I/O#X###USB2PHYCORE_HMAV10GS80.DP
|   Base model USB2PHYCORE_HMAV10GS80
[Model Selector] Selector_11
Model_712 3-STATE,3.3000V,fsdp_tx
Model_714 3-STATE,3.3000V,lsdp_50pf_tx
Model_716 3-STATE,3.3000V,lsdp_200pf_tx
Model_718 3-STATE,3.3000V,lsdp_400pf_tx
Model_720 3-STATE,3.3000V,lsdp_600pf_tx
Model_722 INPUT,3.3V,fsrx
Model_723 3-STATE,0.8000V,hsdp_tx
Model_725 INPUT,3.3V,hsrx
|   Usage OUTPUT#X###USB3_PCIEGEN1_PCIEGEN2_TX.TXP
|   Base model USB3_PCIEGEN1_PCIEGEN2_TX
[Model Selector] Selector_12
Model_500 3-STATE,1.1V,USB3_TX_FS_NO_DEEMPHASIS
Model_501 3-STATE,1.1V,USB3_TX_FS_3p5_DEEMPHASIS
Model_502 3-STATE,1.1V,USB3_TX_HS_NO_DEEMPHASIS
Model_503 3-STATE,1.1V,PCIEGEN1_TX_FS_NO_DEEMPHASIS_1p2v
Model_504 3-STATE,1.1V,PCIEGEN1_TX_FS_NO_DEEMPHASIS_0p8v
Model_505 3-STATE,1.1V,PCIEGEN1_TX_FS_NO_DEEMPHASIS_0p6v
Model_506 3-STATE,1.1V,PCIEGEN1_TX_FS_NO_DEEMPHASIS_0p4v
Model_507 3-STATE,1.1V,PCIEGEN1_TX_FS_3p5_DEEMPHASIS_1p2v
Model_508 3-STATE,1.1V,PCIEGEN1_TX_FS_3p5_DEEMPHASIS_0p8v
Model_509 3-STATE,1.1V,PCIEGEN1_TX_FS_3p5_DEEMPHASIS_0p6v
Model_510 3-STATE,1.1V,PCIEGEN1_TX_FS_3p5_DEEMPHASIS_0p4v
Model_511 3-STATE,1.1V,PCIEGEN1_TX_HS_NO_DEEMPHASIS_0p6v
Model_512 3-STATE,1.1V,PCIEGEN1_TX_HS_NO_DEEMPHASIS_0p4v
Model_513 3-STATE,1.1V,PCIEGEN1_TX_HS_NO_DEEMPHASIS_0p3v
Model_514 3-STATE,1.1V,PCIEGEN1_TX_HS_NO_DEEMPHASIS_0p2v
Model_515 3-STATE,1.1V,PCIEGEN2_TX_FS_NO_DEEMPHASIS_1p2v
Model_516 3-STATE,1.1V,PCIEGEN2_TX_FS_NO_DEEMPHASIS_0p8v
Model_517 3-STATE,1.1V,PCIEGEN2_TX_FS_NO_DEEMPHASIS_0p6v
Model_518 3-STATE,1.1V,PCIEGEN2_TX_FS_NO_DEEMPHASIS_0p4v
Model_519 3-STATE,1.1V,PCIEGEN2_TX_FS_3p5_DEEMPHASIS_1p2v
Model_520 3-STATE,1.1V,PCIEGEN2_TX_FS_3p5_DEEMPHASIS_0p8v
Model_521 3-STATE,1.1V,PCIEGEN2_TX_FS_3p5_DEEMPHASIS_0p6v
Model_522 3-STATE,1.1V,PCIEGEN2_TX_FS_3p5_DEEMPHASIS_0p4v
Model_523 3-STATE,1.1V,PCIEGEN2_TX_FS_6p0_DEEMPHASIS_1p2v
Model_524 3-STATE,1.1V,PCIEGEN2_TX_FS_6p0_DEEMPHASIS_0p8v
Model_525 3-STATE,1.1V,PCIEGEN2_TX_FS_6p0_DEEMPHASIS_0p6v
Model_526 3-STATE,1.1V,PCIEGEN2_TX_FS_6p0_DEEMPHASIS_0p4v
Model_527 3-STATE,1.1V,PCIEGEN2_TX_HS_NO_DEEMPHASIS_0p6v
Model_528 3-STATE,1.1V,PCIEGEN2_TX_HS_NO_DEEMPHASIS_0p4v
Model_529 3-STATE,1.1V,PCIEGEN2_TX_HS_NO_DEEMPHASIS_0p3v
Model_530 3-STATE,1.1V,PCIEGEN2_TX_HS_NO_DEEMPHASIS_0p2v
|   Usage I/O#1.35/1.5/1.8###DDR_DIFFIOPB_H.PADN
|   Base model DDR_DIFFIOPB_H
[Model Selector] Selector_13
Model_413 I/O,1.8V,SR011_DRV48_1P8
Model_414 I/O,1.8V,SR010_DRV48_1P8
Model_415 I/O,1.8V,SR101_DRV48_1P8
Model_416 I/O,1.8V,SR100_DRV48_1P8
Model_417 I/O,1.8V,SR110_DRV48_1P8
Model_418 I/O,1.8V,SR111_DRV48_1P8
Model_419 I/O,1.8V,SR001_DRV48_1P8
Model_420 I/O,1.8V,SR000_DRV48_1P8
Model_421 I/O,1.8V,SR011_DRV40_1P8
Model_422 I/O,1.8V,SR010_DRV40_1P8
Model_423 I/O,1.8V,SR101_DRV40_1P8
Model_424 I/O,1.8V,SR100_DRV40_1P8
Model_425 I/O,1.8V,SR110_DRV40_1P8
Model_426 I/O,1.8V,SR111_DRV40_1P8
Model_427 I/O,1.8V,SR001_DRV40_1P8
Model_428 I/O,1.8V,SR000_DRV40_1P8
Model_429 I/O,1.8V,SR011_DRV34_1P8
Model_430 I/O,1.8V,SR010_DRV34_1P8
Model_431 I/O,1.8V,SR101_DRV34_1P8
Model_432 I/O,1.8V,SR100_DRV34_1P8
Model_433 I/O,1.8V,SR110_DRV34_1P8
Model_434 I/O,1.8V,SR111_DRV34_1P8
Model_435 I/O,1.8V,SR001_DRV34_1P8
Model_436 I/O,1.8V,SR000_DRV34_1P8
Model_437 INPUT,1.5V,DDR3_ODT_80_1P5
Model_438 INPUT,1.5V,DDR3_ODT_60_1P5
Model_439 INPUT,1.5V,DDR3_ODT_120_1P5
Model_440 INPUT,1.35V,DDR3L_ODT_80_1P35
Model_441 INPUT,1.35V,DDR3L_ODT_60_1P35
Model_442 INPUT,1.35V,DDR3L_ODT_120_1P35
Model_443 INPUT,1.8V,DDR2_ODT_120_1P8
Model_444 INPUT,1.8V,DDR2_ODT_80_1P8
Model_445 INPUT,1.8V,DDR2_ODT_60_1P8
Model_446 I/O,1.5V,SR011_DRV40_1P5
Model_447 I/O,1.5V,SR010_DRV40_1P5
Model_448 I/O,1.5V,SR101_DRV40_1P5
Model_449 I/O,1.5V,SR100_DRV40_1P5
Model_450 I/O,1.5V,SR110_DRV40_1P5
Model_451 I/O,1.5V,SR111_DRV40_1P5
Model_452 I/O,1.5V,SR001_DRV40_1P5
Model_453 I/O,1.5V,SR000_DRV40_1P5
Model_454 I/O,1.5V,SR011_DRV34_1P5
Model_455 I/O,1.5V,SR010_DRV34_1P5
Model_456 I/O,1.5V,SR101_DRV34_1P5
Model_457 I/O,1.5V,SR100_DRV34_1P5
Model_458 I/O,1.5V,SR110_DRV34_1P5
Model_459 I/O,1.5V,SR111_DRV34_1P5
Model_460 I/O,1.5V,SR001_DRV34_1P5
Model_461 I/O,1.5V,SR000_DRV34_1P5
Model_462 I/O,1.5V,SR011_DRV48_1P5
Model_463 I/O,1.5V,SR010_DRV48_1P5
Model_464 I/O,1.5V,SR101_DRV48_1P5
Model_465 I/O,1.5V,SR100_DRV48_1P5
Model_466 I/O,1.5V,SR110_DRV48_1P5
Model_467 I/O,1.5V,SR111_DRV48_1P5
Model_468 I/O,1.5V,SR001_DRV48_1P5
Model_469 I/O,1.5V,SR000_DRV48_1P5
Model_470 I/O,1.35V,SR011_DRV40_1P35
Model_471 I/O,1.35V,SR010_DRV40_1P35
Model_472 I/O,1.35V,SR101_DRV40_1P35
Model_473 I/O,1.35V,SR100_DRV40_1P35
Model_474 I/O,1.35V,SR110_DRV40_1P35
Model_475 I/O,1.35V,SR111_DRV40_1P35
Model_476 I/O,1.35V,SR001_DRV40_1P35
Model_477 I/O,1.35V,SR000_DRV40_1P35
Model_478 I/O,1.35V,SR011_DRV34_1P35
Model_479 I/O,1.35V,SR010_DRV34_1P35
Model_480 I/O,1.35V,SR101_DRV34_1P35
Model_481 I/O,1.35V,SR100_DRV34_1P35
Model_482 I/O,1.35V,SR110_DRV34_1P35
Model_483 I/O,1.35V,SR111_DRV34_1P35
Model_484 I/O,1.35V,SR001_DRV34_1P35
Model_485 I/O,1.35V,SR000_DRV34_1P35
Model_486 I/O,1.35V,SR011_DRV48_1P35
Model_487 I/O,1.35V,SR010_DRV48_1P35
Model_488 I/O,1.35V,SR101_DRV48_1P35
Model_489 I/O,1.35V,SR100_DRV48_1P35
Model_490 I/O,1.35V,SR110_DRV48_1P35
Model_491 I/O,1.35V,SR111_DRV48_1P35
Model_492 I/O,1.35V,SR001_DRV48_1P35
Model_493 I/O,1.35V,SR000_DRV48_1P35
|   Usage OUTPUT#1.35/1.5/1.8###DDR_DIFFIOPB_V.PADP
|   Base model DDR_DIFFIOPB_V
[Model Selector] Selector_14
Model_618 I/O,1.8V,SR011_DRV48_1P8
Model_619 I/O,1.8V,SR010_DRV48_1P8
Model_620 I/O,1.8V,SR101_DRV48_1P8
Model_621 I/O,1.8V,SR100_DRV48_1P8
Model_622 I/O,1.8V,SR110_DRV48_1P8
Model_623 I/O,1.8V,SR111_DRV48_1P8
Model_624 I/O,1.8V,SR001_DRV48_1P8
Model_625 I/O,1.8V,SR000_DRV48_1P8
Model_626 I/O,1.8V,SR011_DRV40_1P8
Model_627 I/O,1.8V,SR010_DRV40_1P8
Model_628 I/O,1.8V,SR101_DRV40_1P8
Model_629 I/O,1.8V,SR100_DRV40_1P8
Model_630 I/O,1.8V,SR110_DRV40_1P8
Model_631 I/O,1.8V,SR111_DRV40_1P8
Model_632 I/O,1.8V,SR001_DRV40_1P8
Model_633 I/O,1.8V,SR000_DRV40_1P8
Model_634 I/O,1.8V,SR011_DRV34_1P8
Model_635 I/O,1.8V,SR010_DRV34_1P8
Model_636 I/O,1.8V,SR101_DRV34_1P8
Model_637 I/O,1.8V,SR100_DRV34_1P8
Model_638 I/O,1.8V,SR110_DRV34_1P8
Model_639 I/O,1.8V,SR111_DRV34_1P8
Model_640 I/O,1.8V,SR001_DRV34_1P8
Model_641 I/O,1.8V,SR000_DRV34_1P8
Model_651 I/O,1.5V,SR011_DRV40_1P5
Model_652 I/O,1.5V,SR010_DRV40_1P5
Model_653 I/O,1.5V,SR101_DRV40_1P5
Model_654 I/O,1.5V,SR100_DRV40_1P5
Model_655 I/O,1.5V,SR110_DRV40_1P5
Model_656 I/O,1.5V,SR111_DRV40_1P5
Model_657 I/O,1.5V,SR001_DRV40_1P5
Model_658 I/O,1.5V,SR000_DRV40_1P5
Model_659 I/O,1.5V,SR011_DRV34_1P5
Model_660 I/O,1.5V,SR010_DRV34_1P5
Model_661 I/O,1.5V,SR101_DRV34_1P5
Model_662 I/O,1.5V,SR100_DRV34_1P5
Model_663 I/O,1.5V,SR110_DRV34_1P5
Model_664 I/O,1.5V,SR111_DRV34_1P5
Model_665 I/O,1.5V,SR001_DRV34_1P5
Model_666 I/O,1.5V,SR000_DRV34_1P5
Model_667 I/O,1.5V,SR011_DRV48_1P5
Model_668 I/O,1.5V,SR010_DRV48_1P5
Model_669 I/O,1.5V,SR101_DRV48_1P5
Model_670 I/O,1.5V,SR100_DRV48_1P5
Model_671 I/O,1.5V,SR110_DRV48_1P5
Model_672 I/O,1.5V,SR111_DRV48_1P5
Model_673 I/O,1.5V,SR001_DRV48_1P5
Model_674 I/O,1.5V,SR000_DRV48_1P5
Model_675 I/O,1.35V,SR011_DRV40_1P35
Model_676 I/O,1.35V,SR010_DRV40_1P35
Model_677 I/O,1.35V,SR101_DRV40_1P35
Model_678 I/O,1.35V,SR100_DRV40_1P35
Model_679 I/O,1.35V,SR110_DRV40_1P35
Model_680 I/O,1.35V,SR111_DRV40_1P35
Model_681 I/O,1.35V,SR001_DRV40_1P35
Model_682 I/O,1.35V,SR000_DRV40_1P35
Model_683 I/O,1.35V,SR011_DRV34_1P35
Model_684 I/O,1.35V,SR010_DRV34_1P35
Model_685 I/O,1.35V,SR101_DRV34_1P35
Model_686 I/O,1.35V,SR100_DRV34_1P35
Model_687 I/O,1.35V,SR110_DRV34_1P35
Model_688 I/O,1.35V,SR111_DRV34_1P35
Model_689 I/O,1.35V,SR001_DRV34_1P35
Model_690 I/O,1.35V,SR000_DRV34_1P35
Model_691 I/O,1.35V,SR011_DRV48_1P35
Model_692 I/O,1.35V,SR010_DRV48_1P35
Model_693 I/O,1.35V,SR101_DRV48_1P35
Model_694 I/O,1.35V,SR100_DRV48_1P35
Model_695 I/O,1.35V,SR110_DRV48_1P35
Model_696 I/O,1.35V,SR111_DRV48_1P35
Model_697 I/O,1.35V,SR001_DRV48_1P35
Model_698 I/O,1.35V,SR000_DRV48_1P35
|   Usage I/O#1.35/1.5/1.8###DDR_SEIOPB_H.PAD
|   Base model DDR_SEIOPB_H
[Model Selector] Selector_15
Model_242 I/O,1.8V,SR011_DRV48_1P8
Model_243 I/O,1.8V,SR010_DRV48_1P8
Model_244 I/O,1.8V,SR101_DRV48_1P8
Model_245 I/O,1.8V,SR100_DRV48_1P8
Model_246 I/O,1.8V,SR110_DRV48_1P8
Model_247 I/O,1.8V,SR111_DRV48_1P8
Model_248 I/O,1.8V,SR001_DRV48_1P8
Model_249 I/O,1.8V,SR000_DRV48_1P8
Model_250 I/O,1.8V,SR011_DRV40_1P8
Model_251 I/O,1.8V,SR010_DRV40_1P8
Model_252 I/O,1.8V,SR101_DRV40_1P8
Model_253 I/O,1.8V,SR100_DRV40_1P8
Model_254 I/O,1.8V,SR110_DRV40_1P8
Model_255 I/O,1.8V,SR111_DRV40_1P8
Model_256 I/O,1.8V,SR001_DRV40_1P8
Model_257 I/O,1.8V,SR000_DRV40_1P8
Model_258 I/O,1.8V,SR011_DRV34_1P8
Model_259 I/O,1.8V,SR010_DRV34_1P8
Model_260 I/O,1.8V,SR101_DRV34_1P8
Model_261 I/O,1.8V,SR100_DRV34_1P8
Model_262 I/O,1.8V,SR110_DRV34_1P8
Model_263 I/O,1.8V,SR111_DRV34_1P8
Model_264 I/O,1.8V,SR001_DRV34_1P8
Model_265 I/O,1.8V,SR000_DRV34_1P8
Model_266 INPUT,1.5V,DDR3_ODT_80_1P5
Model_267 INPUT,1.5V,DDR3_ODT_60_1P5
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| Models and submodels in the file (398): Model_81 (I/O), Model_82 (I/O), Model_83 (I/O), Model_84 (I/O), Model_85 (I/O), Model_86 (I/O), Model_87 (I/O), Model_88 (I/O), Model_89 (I/O), Model_90 (I/O), Model_91 (I/O), Model_92 (I/O), Model_93 (I/O), Model_94 (I/O), Model_95 (I/O), Model_96 (I/O), Model_97 (I/O), Model_98 (I/O), Model_99 (I/O), Model_100 (I/O), Model_101 (I/O), Model_102 (I/O), Model_103 (I/O), Model_104 (I/O), Model_114 (I/O), Model_115 (I/O), Model_116 (I/O), Model_117 (I/O), Model_118 (I/O), Model_119 (I/O), Model_120 (I/O), Model_121 (I/O), Model_122 (I/O), Model_123 (I/O), Model_124 (I/O), Model_125 (I/O), Model_126 (I/O), Model_127 (I/O), Model_128 (I/O), Model_129 (I/O), Model_130 (I/O), Model_131 (I/O), Model_132 (I/O), Model_133 (I/O), Model_134 (I/O), Model_135 (I/O), Model_136 (I/O), Model_137 (I/O), Model_138 (I/O), Model_139 (I/O), Model_140 (I/O), Model_141 (I/O), Model_142 (I/O), Model_143 (I/O), Model_144 (I/O), Model_145 (I/O), Model_146 (I/O), Model_147 (I/O), Model_148 (I/O), Model_149 (I/O), Model_150 (I/O), Model_151 (I/O), Model_152 (I/O), Model_153 (I/O), Model_154 (I/O), Model_155 (I/O), Model_156 (I/O), Model_157 (I/O), Model_158 (I/O), Model_159 (I/O), Model_160 (I/O), Model_161 (I/O), Model_242 (I/O), Model_243 (I/O), Model_244 (I/O), Model_245 (I/O), Model_246 (I/O), Model_247 (I/O), Model_248 (I/O), Model_249 (I/O)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
